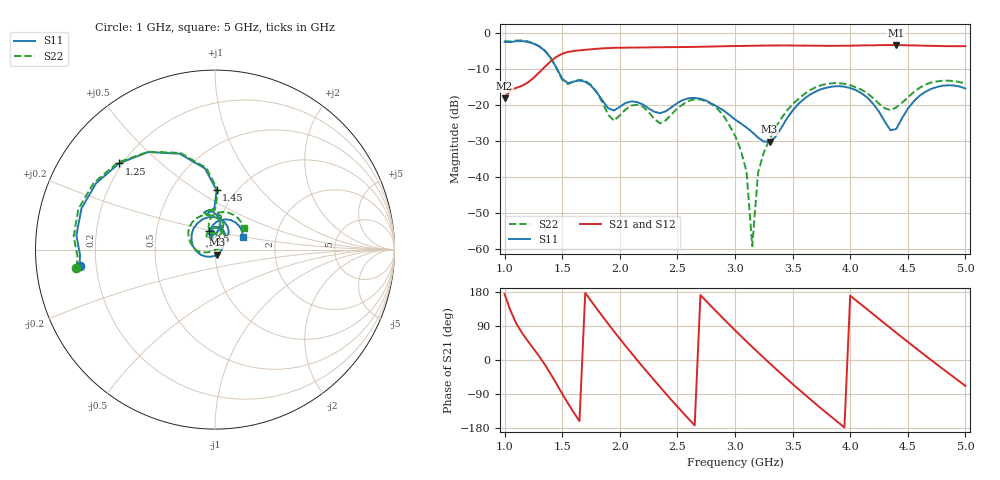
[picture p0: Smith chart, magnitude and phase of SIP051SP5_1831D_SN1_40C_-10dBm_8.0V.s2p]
# GHz  S  dB  R  50
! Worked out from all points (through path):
!   81 points, 1 GHz to 5 GHz, reference 50 ohm
!   highest |S21| = -3.28 dB at 4.4 GHz (marker M1); lowest = -18.1 dB at 1 GHz (marker M2)
!   lowest |S11| = -30.1 dB at 3.3 GHz (marker M3), VSWR 1.06, Z = 51.3 - j2.87 ohm
!   |S11| at or under -10 dB: 1.457 GHz to end of sweep
!   |S22| runs from -59.1 to -2.0 dB; largest |S21 - S12| = 0.0027
!   S11 on the Smith chart (normalised r, x): 1 GHz: 0.14, -0.06; 1.25 GHz: 0.19, +0.37; 1.45 GHz: 0.82, +0.61; 2.5 GHz: 0.92, +0.19; 5 GHz: 1.35, +0.20
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1  -2.38 -173.2  -18.08 173.9  -18.09 174.1  -2.17 -172.6
1.25  -2.87 138.1  -12.43 30.4  -12.45 30.6  -2.77 138.1
1.45  -9.60 88.4  -6.54 -62.7  -6.52 -62.7  -9.68 87.1
1.55  -13.87 102.3  -5.20 -114.4  -5.19 -114.5  -14.10 102.4
1.7  -13.47 93.5  -4.59 177.1  -4.60 177.1  -13.19 91.6
1.95  -21.45 100.8  -4.05 75.4  -4.06 75.4  -24.30 99.7
2.15  -19.12 97.8  -3.97 0.0  -3.96 -0.0  -19.87 99.6
2.35  -22.20 102.9  -3.89 -71.4  -3.88 -71.4  -25.00 103.6
2.5  -19.35 107.8  -3.85 -123.0  -3.86 -123.0  -20.86 121.7
2.7  -18.20 75.3  -3.75 171.4  -3.76 171.4  -18.38 84.1
3  -23.93 34.3  -3.54 78.5  -3.55 78.6  -28.40 24.1
3.1  -26.18 21.2  -3.50 48.9  -3.50 49.0  -38.38 5.6
3.15  -27.46 10.5  -3.48 34.4  -3.48 34.4  -59.12 -101.1
3.2  -28.97 -4.9  -3.45 20.0  -3.46 20.0  -38.74 -156.4
3.3  -30.14 -63.9  -3.41 -8.3  -3.40 -8.4  -29.50 -158.3
3.5  -21.47 -160.1  -3.41 -63.3  -3.41 -63.3  -19.70 -177.8
3.7  -16.18 147.1  -3.47 -115.7  -3.47 -115.6  -15.00 147.0
4  -15.21 81.1  -3.46 169.8  -3.47 169.6  -14.43 94.3
4.35  -26.93 64.1  -3.29 84.1  -3.30 84.1  -21.37 90.5
4.4  -26.57 93.9  -3.29 71.9  -3.28 71.8  -20.60 100.8
4.7  -15.49 79.5  -3.49 0.5  -3.49 0.6  -13.71 85.9
5  -15.33 24.9  -3.58 -68.4  -3.59 -68.4  -13.96 36.3
